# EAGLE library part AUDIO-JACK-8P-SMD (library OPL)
When you use the footprint ,place notice 46 (layer)milling ,there is some important information.
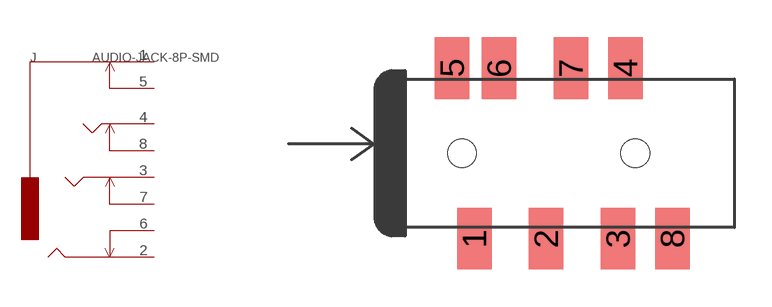
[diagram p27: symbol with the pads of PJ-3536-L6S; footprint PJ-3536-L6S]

Designator prefix J

## AUDIO-JACK-8P-SMD-320040003  [PJ-3536-L6S]
1  1
2  2
3  3
4  4
5  5
6  6
7  7
8  8

## Footprint PJ-3536-L6S (pad centres in mm)
smd 1.4 x 2.5: 1 2.8,-3.45; 2 5.7,-3.45; 3 8.6,-3.45; 4 8.9,3.45; 5 1.9,3.45; 6 3.8,3.45; 7 6.7,3.45; 8 10.8,-3.45
hole 1.149 at 2.3,0
hole 1.149 at 9.3,0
